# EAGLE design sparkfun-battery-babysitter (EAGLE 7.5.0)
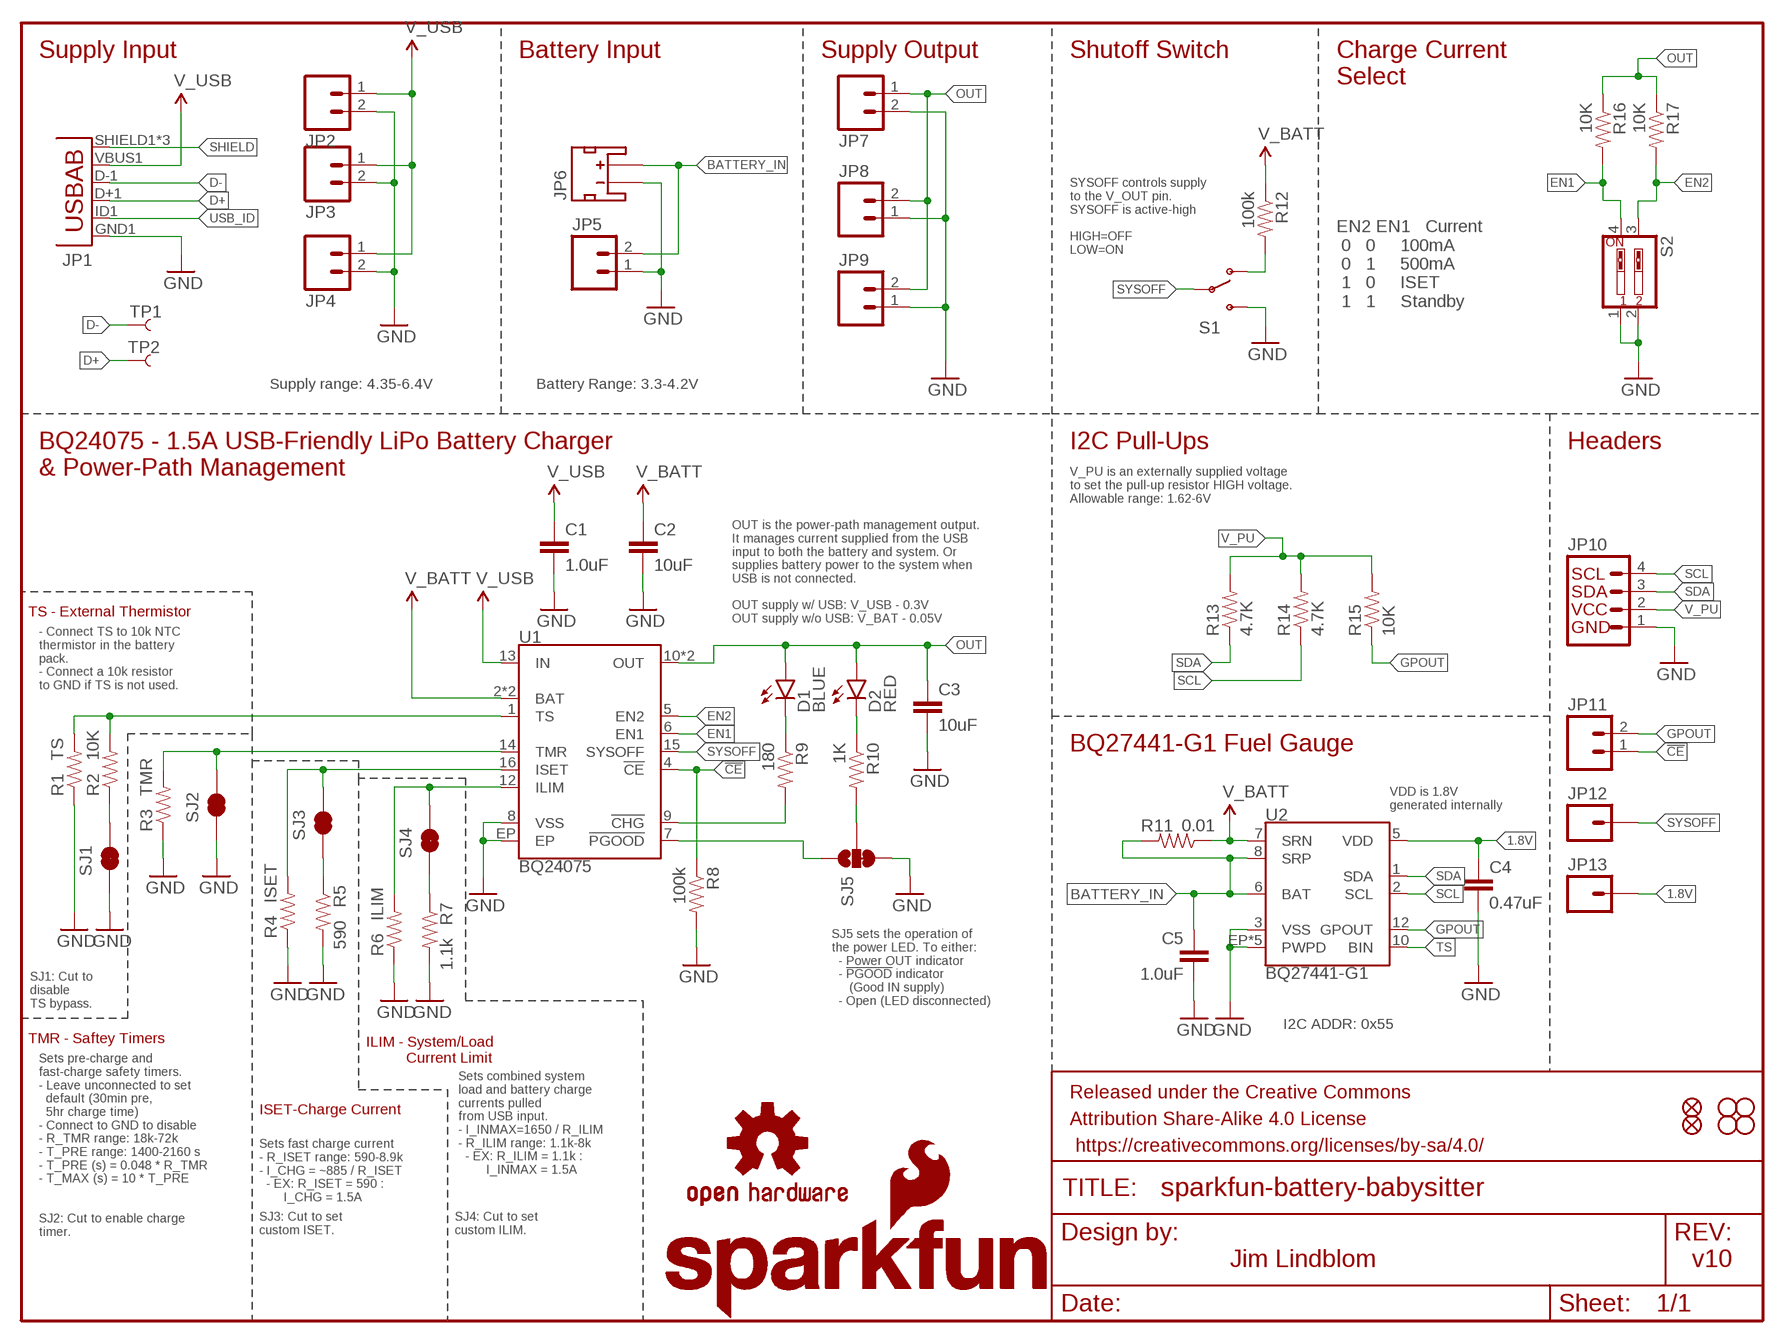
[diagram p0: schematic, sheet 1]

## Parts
C1  1.0uF  1.0UF50V10%(1206)  [1206-CAP]
C2  10uF  10UF10V10%(0805)  [0805-CAP]
C3  10uF  10UF10V10%(0805)  [0805-CAP]
C4  0.47uF  CAP0603-CAP  [0603-CAP]
C5  1.0uF  1.0UF-16V-10%(0603)  [0603-CAP]
D1  BLUE  LED-BLUE0603  [LED-0603]
D2  RED  LED-RED0603  [LED-0603]
FID1  FIDUCIAL1X2  [FIDUCIAL-1X2]
FID2  FIDUCIAL1X2  [FIDUCIAL-1X2]
FRAME1  FRAME-LETTER  [CREATIVE_COMMONS]
JP1  USB-ABCONN-11794  [USB-AB-MICRO-SMD_V03]
JP2  M021X02_NO_SILK  [1X02_NO_SILK]
JP3  M023.5MM-NO_SILK  [SCREWTERMINAL-3.5MM-2-NS]
JP4  M021X02_NO_SILK  [1X02_NO_SILK]
JP5  M021X02_NO_SILK  [1X02_NO_SILK]
JP6  JST_2MM_MALE  [JST-2-SMD]
JP7  M023.5MM-NO_SILK  [SCREWTERMINAL-3.5MM-2-NS]
JP8  M021X02_NO_SILK  [1X02_NO_SILK]
JP9  M02-JST-2-PTH-NO_SILK  [JST-2-PTH-NS]
JP10  I2C_STANDARD_NO_SILK  [1X04_NO_SILK]
JP11  M021X02_NO_SILK  [1X02_NO_SILK]
JP12  M01PTH_NO_SILK_YES_STOP  [1X01_NO_SILK]
JP13  M01PTH_NO_SILK_YES_STOP  [1X01_NO_SILK]
LOGO1  SFE_LOGO_NAME.1_INCH  [SFE_LOGO_NAME_.1]
LOGO2  SFE_LOGO_NAME_FLAME.1_INCH  [SFE_LOGO_NAME_FLAME_.1]
LOGO3  OSHW-LOGOS  [OSHW-LOGO-S]
R1  TS  RESISTORPTH-1/6W  [1/6W-RES]
R2  10K  10KOHM-1/10W-1%(0603)0603  [0603-RES]
R3  TMR  RESISTORPTH-1/6W  [1/6W-RES]
R4  ISET  RESISTORPTH-1/6W  [1/6W-RES]
R5  590  RESISTOR0603-RES  [0603-RES]
R6  ILIM  RESISTORPTH-1/6W  [1/6W-RES]
R7  1.1k  RESISTOR0603-RES  [0603-RES]
R8  100k  100KOHM-1/10W-1%(0603)  [0603-RES]
R9  180  180OHM1/10W1%(0603)  [0603-RES]
R10  1K  1KOHM-1/10W-1%(0603)  [0603-RES]
R11  0.01  RESISTOR1206  [1206]
R12  100k  100KOHM-1/10W-1%(0603)  [0603-RES]
R13  4.7K  4.7KOHM-1/10W-1%(0603)  [0603-RES]
R14  4.7K  4.7KOHM-1/10W-1%(0603)  [0603-RES]
R15  10K  10KOHM-1/10W-1%(0603)0603  [0603-RES]
R16  10K  10KOHM-1/10W-1%(0603)0603  [0603-RES]
R17  10K  10KOHM-1/10W-1%(0603)0603  [0603-RES]
S1  SWITCH-SPDT-SMD-A  [SWITCH-SPST-SMD-A]
S2  SW_DIP-2-SMT-HALFSIZE  [DIPSWITCH-02-50MIL]
SJ1  JUMPER-PAD-2-NC_BY_TRACE  [PAD-JUMPER-2-NC_BY_TRACE_YES_SILK]
SJ2  JUMPER-PAD-2-NC_BY_TRACE  [PAD-JUMPER-2-NC_BY_TRACE_YES_SILK]
SJ3  JUMPER-PAD-2-NC_BY_TRACE  [PAD-JUMPER-2-NC_BY_TRACE_YES_SILK]
SJ4  JUMPER-PAD-2-NC_BY_TRACE  [PAD-JUMPER-2-NC_BY_TRACE_YES_SILK]
SJ5  JUMPER-PAD-3-2OF3_NC_BY_TRACE_SMALL  [PAD-JUMPER-3-2OF3_NC_BY_TRACE_YES_SILK_FULL_BOX]
STANDOFF1  STAND-OFF  [STAND-OFF]
STANDOFF2  STAND-OFF  [STAND-OFF]
STANDOFF3  STAND-OFF  [STAND-OFF]
STANDOFF4  STAND-OFF  [STAND-OFF]
TP1  TEST-POINT3X4  [PAD.03X.04]
TP2  TEST-POINT3X4  [PAD.03X.04]
U1  BQ24075  [PVQFN-N16]
U2  BQ27441-G1  [PDSO-N12]

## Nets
1.8V: C4.1 JP13.1 U2.5(VDD)
!CE!: JP11.1 R8.1 U1.4(!CE!)
!CHG!: R9.2 U1.9(!CHG!)
!PGOOD!: SJ5.1 U1.7(!PGOOD!)
BATTERY_IN: C5.1 JP5.2 JP6.2(+) R11.2 U2.6(BAT) U2.8(SRP)
D+: JP1.D+1(D+) TP2.P$1
D-: JP1.D-1(D-) TP1.P$1
EN1: R16.2 S2.4 U1.6(EN1)
EN2: R17.2 S2.3 U1.5(EN2)
GND: C1.2 C2.2 C3.2 C4.2 C5.2 JP1.GND1(GND) JP2.2 JP3.2 JP4.2 JP5.1 JP6.1(-) JP7.2 JP8.1 JP9.1 JP10.1 R1.1 R3.1 R4.1 R5.2 R6.1 R7.2 R8.2 S1.3(S) S2.1 S2.2 SJ1.1 SJ2.1 SJ5.3 U1.8(VSS) U1.EP U2.3(VSS) U2.EP1(PWPD) U2.EP2(PWPD) U2.EP3(PWPD) U2.EP4(PWPD) U2.EP(PWPD)
GPOUT: JP11.2 R15.1 U2.12(GPOUT)
ILIM: R6.2 SJ4.2 U1.12(ILIM)
ISET: R4.2 SJ3.2 U1.16(ISET)
N$1: R2.1 SJ1.2
N$2: R7.1 SJ4.1
N$3: R5.1 SJ3.1
N$4: R12.2 S1.1(O)
N$5: R10.2 SJ5.2
N$11: D1.C R9.1
N$12: D2.C R10.1
OUT: C3.1 D1.A D2.A JP7.1 JP8.2 JP9.2 R16.1 R17.1 U1.10(OUT) U1.11(OUT)
SCL: JP10.4 R14.1 U2.2(SCL)
SDA: JP10.3 R13.1 U2.1(SDA)
SHIELD: JP1.SHIELD1(SHIELD) JP1.SHIELD2(SHIELD) JP1.SHIELD3(SHIELD)
SYSOFF: JP12.1 S1.2(P) U1.15(SYSOFF)
TMR: R3.2 SJ2.2 U1.14(TMR)
TS: R1.2 R2.2 U1.1(TS) U2.10(BIN)
USB_ID: JP1.ID1(USBID)
V_BATT: C2.1 R11.1 R12.1 U1.2(BAT) U1.3(BAT) U2.7(SRN)
V_PU: JP10.2 R13.2 R14.2 R15.2
V_USB: C1.1 JP1.VBUS1(VBUS) JP2.1 JP3.1 JP4.1 U1.13(IN)
Unconnected: JP6.NC1(PAD1) JP6.NC2(PAD2)

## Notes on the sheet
- Supply Input | Battery Input | Supply Output | Shutoff Switch
- Charge Current
  Select
- SYSOFF controls supply 
  to the V_OUT pin.
  SYSOFF is active-high
  
  HIGH=OFF
  LOW=ON
- EN2 EN1   Current
   0   0     100mA
   0   1     500mA
   1   0     ISET
   1   1     Standby
- Supply range: 4.35-6.4V | Battery Range: 3.3-4.2V
- BQ24075 - 1.5A USB-Friendly LiPo Battery Charger 
  & Power-Path Management
- I2C Pull-Ups | Headers
- V_PU is an externally supplied voltage 
  to set the pull-up resistor HIGH voltage.
  Allowable range: 1.62-6V
- OUT is the power-path management output.
  It manages current supplied from the USB 
  input to both the battery and system. Or
  supplies battery power to the system when 
  USB is not connected.
  
  OUT supply w/ USB: V_USB - 0.3V
  OUT supply w/o USB: V_BAT - 0.05V
- TS - External Thermistor
- - Connect TS to 10k NTC 
  thermistor in the battery
  pack.
  - Connect a 10k resistor 
  to GND if TS is not used.
- BQ27441-G1 Fuel Gauge
- VDD is 1.8V
  generated internally
- SJ5 sets the operation of 
  the power LED. To either:
    - Power OUT indicator
    - !PGOOD! indicator 
       (Good IN supply)
    - Open (LED disconnected)
- SJ1: Cut to 
  disable
  TS bypass.
- I2C ADDR: 0x55
- TMR - Saftey Timers
- ILIM - System/Load 
            Current Limit
- Sets pre-charge and
  fast-charge safety timers.
  - Leave unconnected to set
    default (30min pre, 
    5hr charge time)
  - Connect to GND to disable
  - R_TMR range: 18k-72k
  - T_PRE range: 1400-2160 s
  - T_PRE (s) = 0.048 * R_TMR
  - T_MAX (s) = 10 * T_PRE
- Sets combined system
  load and battery charge 
  currents pulled
  from USB input.
  - I_INMAX=1650 / R_ILIM
  - R_ILIM range: 1.1k-8k
    - EX: R_ILIM = 1.1k : 
          I_INMAX = 1.5A
- ISET-Charge Current
- Sets fast charge current
  - R_ISET range: 590-8.9k
  - I_CHG = ~885 / R_ISET
    - EX: R_ISET = 590 : 
         I_CHG = 1.5A
- SJ3: Cut to set
  custom ISET.
- SJ4: Cut to set
  custom ILIM.
- SJ2: Cut to enable charge
  timer.
- Jim Lindblom | v10

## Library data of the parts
C1 = SparkFun-Capacitors:1.0UF50V10%(1206): CAP-09822; PROD_ID: CAP-09822
C2 C3 = SparkFun-Capacitors:10UF10V10%(0805): CAP-11330; PROD_ID: CAP-11330
C4 = SparkFun-Capacitors:CAP: Capacitor; PROD_ID: CAP-13216
C5 = SparkFun-Capacitors:1.0UF-16V-10%(0603): CAP-00868; PROD_ID: CAP-00868
D1 = SparkFun-LED:LED-BLUE: Blue LEDs for production use; PROD_ID: DIO-08575
D2 = SparkFun-LED:LED-RED: Assorted Red LEDs; PROD_ID: DIO-00819
FID1 FID2 = SparkFun-Aesthetics:FIDUCIAL: Fiducial Alignment Points
FRAME1 = SparkFun-Aesthetics:FRAME-LETTER: Schematic Frame
JP1 = SparkFun-Connectors:USB-AB: This is a USB AB connector that is compatible with USB OTG. i.e. this connector can serve as a host or device; PROD_ID: CONN-11794
JP2 JP4 JP5 JP8 JP9 JP11 = SparkFun-Connectors:M02: Standard 2-pin 0.1" header. Use with
JP3 JP7 = SparkFun-Connectors:M02: Standard 2-pin 0.1" header. Use with; PROD_ID: CONN-08399
JP6 = SparkFun-Connectors:JST_2MM_MALE: Mates to single-cell LiPo batteries. CONN-11443 Now with smashable polarity marks!; BTM_NEG: -; BTM_POS: +; PROD_ID: CONN-11443; TOP_NEG: -; TOP_POS: +
JP10 = SparkFun-Connectors:I2C_STANDARD: SparkFun has standardized on a pinout for all I2C based sensor breakouts. This pinout allows I2C boards to be plugged directly into the headers on Arduino Uno compatible boards, and to be daisy chained easily.
JP12 JP13 = SparkFun-Connectors:M01: Header 1
LOGO1 = SparkFun-Aesthetics:SFE_LOGO_NAME: SFE Logo, name only
LOGO2 = SparkFun-Aesthetics:SFE_LOGO_NAME_FLAME: SFE Logo, name and flame
LOGO3 = SparkFun-Aesthetics:OSHW-LOGO: Open Source Hardware Logo
R1 R3 R4 R6 = SparkFun-Resistors:RESISTOR: Resistor
R2 R15-R17 = SparkFun-Resistors:10KOHM-1/10W-1%(0603): RES-00824; PROD_ID: RES-00824
R5 = SparkFun-Passives:RESISTOR: Resistor; PROD_ID: RES-13217
R7 = SparkFun-Passives:RESISTOR: Resistor; PROD_ID: RES-10447
R8 R12 = SparkFun-Resistors:100KOHM-1/10W-1%(0603): RES-07828; PROD_ID: RES-07828
R9 = SparkFun-Resistors:180OHM1/10W1%(0603): RES-08788; PROD_ID: RES-08788
R10 = SparkFun-Resistors:1KOHM-1/10W-1%(0603): RES-07856; PROD_ID: RES-07856
R11 = SparkFun-Resistors:RESISTOR: Resistor; PROD_ID: RES-13218
R13 R14 = SparkFun-Resistors:4.7KOHM-1/10W-1%(0603): RES-07857; PROD_ID: RES-07857
S1 = SparkFun-Electromechanical:SWITCH-SPDT: SPDT Switch Simple slide switch, Spark Fun Electronics SKU : COM-00102 DPDT SMT slide switch, AYZ0202, SWCH-08179; PROD_ID: SWCH-10651
S2 = SparkFun-Electromechanical:SW_DIP-2: DIP SWITCH; PROD_ID: SWCH-13215
SJ1-SJ4 = SparkFun-Passives:JUMPER-PAD-2-NC_BY_TRACE
SJ5 = SparkFun-Passives:JUMPER-PAD-3-2OF3_NC_BY_TRACE
STANDOFF1-STANDOFF4 = SparkFun-Electromechanical:STAND-OFF: #4 Stand Off
TP1 TP2 = SparkFun-Passives:TEST-POINT: Bare copper test points for troubleshooting or ICT
U1 = battery-management-temp:BQ24075; PROD_ID: IC-13219
U2 = battery-management-temp:BQ27441-G1; PROD_ID: IC-13220

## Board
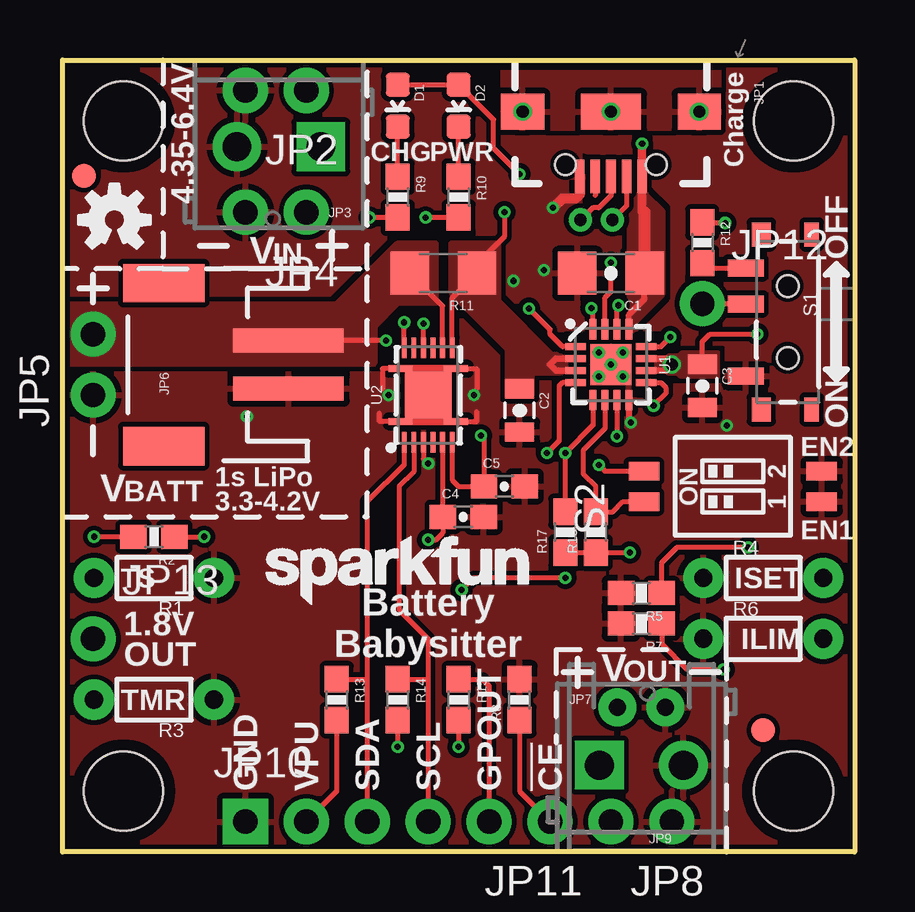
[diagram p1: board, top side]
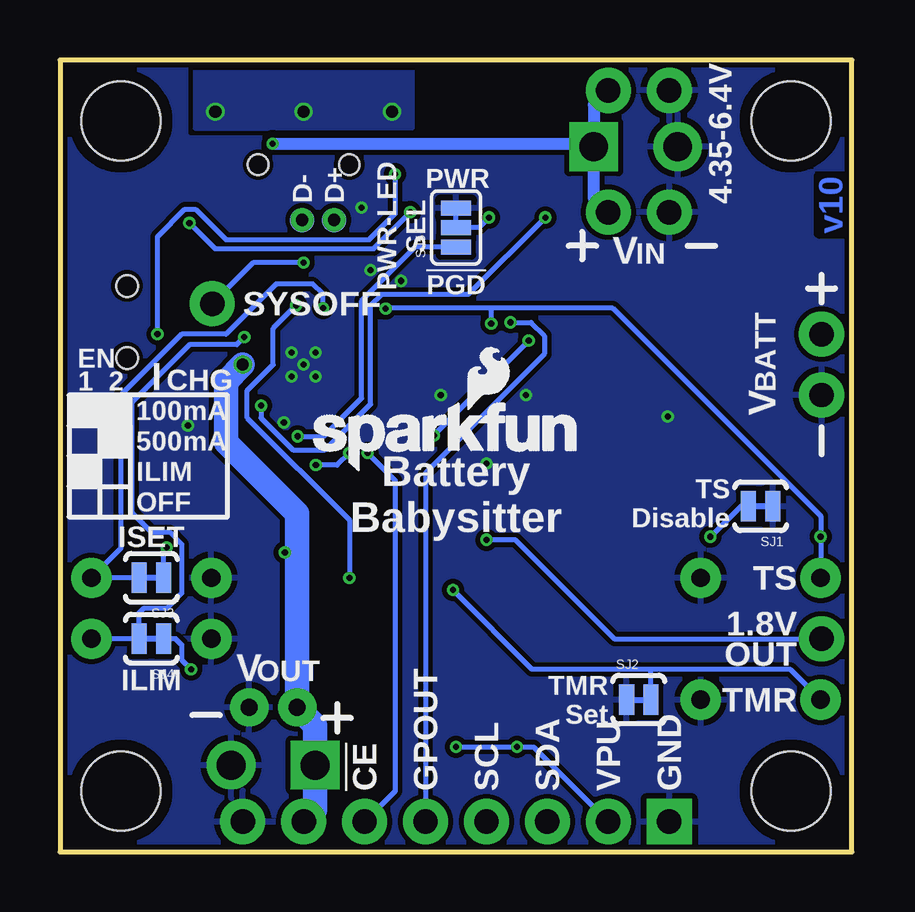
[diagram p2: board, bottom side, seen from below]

Size 33.02 x 33.02 mm. Coordinates in mm from the lower left corner, seen from the top.
Outline: 0,33.02 33.02,33.02 33.02,0 0,0 0,33.02
Copper layers (1*16): Top 0.035mm / dielectric 1.5mm / Bottom 0.035mm
Design rules "SparkFun-2-layer-FAB-LIMIT *": minimum track width 7mil, minimum drill 6mil, track to track 7mil, track to pad 7mil, pad to pad 7mil, via to via 7mil, smd to smd 7mil, copper to edge 7mil, drill to drill 7mil, minimum pad ring 5mil, minimum via ring 5mil, stop-mask expansion 4mil, vias tented up to drill 20mil, thermal gap 10mil

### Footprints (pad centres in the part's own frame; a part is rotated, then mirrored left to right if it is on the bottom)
1206-CAP = smd 1.6 x 1.8: 1 -1.4,0; 2 1.4,0
0805-CAP = smd 0.8 x 1.2: 1 -0.9,0; 2 0.9,0
0603-CAP = smd 1.1 x 1: 1 -0.85,0; 2 0.85,0
LED-0603 = smd 1 x 1: A 0,-0.877; C 0,0.877
FIDUCIAL-1X2 = smd 1 x 1: 1 0,0
USB-AB-MICRO-SMD_V03 = smd 1.4 x 0.4: D+1 2.7,0; D-1 2.7,0.65; GND1 2.7,-1.3; ID1 2.7,-0.65; VBUS1 2.7,1.3 | smd 1.5 x 1.8: SHIELD1 0,3.68; SHIELD3 0,-3.68 | smd 1.5 x 2.5: SHIELD2 0,0 | hole 0.85: 2.2,1.9; 2.2,-1.9
1X02_NO_SILK = drill 1.016 pad 1.88: 1 0,0; 2 2.54,0
SCREWTERMINAL-3.5MM-2-NS = drill 1.2 pad 2.032 square: 1 0,0 | drill 1.2 pad 2.032: 2 3.5,0
JST-2-SMD = smd 1 x 4.6: 1 -1,-3.7; 2 1,-3.7 | smd 1.6 x 3.4: NC1 -3.4,1.5; NC2 3.4,1.5
JST-2-PTH-NS = drill 0.7 pad 1.6: 1 -1,0; 2 1,0
1X04_NO_SILK = drill 1.016 pad 1.88 square: 1 0,0 | drill 1.016 pad 1.88: 2 2.54,0; 3 5.08,0; 4 7.62,0
1X01_NO_SILK = drill 1.016 pad 1.88: 1 0,0
1/6W-RES = drill 0.762 pad 1.676: 1 -2.5,0; 2 2.5,0
0603-RES = smd 1.1 x 1: 1 -0.85,0; 2 0.85,0
1206 = smd 1.6 x 1.8: 1 -1.4,0; 2 1.4,0
SWITCH-SPST-SMD-A = smd 0.7 x 1.5: 1 -2.25,-1.75; 2 -0.75,-1.75; 3 2.25,-1.75 | smd 1 x 0.6: GND1 -3.65,1; GND3 3.65,1 | smd 1 x 0.8: GND2 -3.65,-1.1; GND4 3.65,-1.1 | hole 0.9: -1.5,0; 1.5,0
DIPSWITCH-02-50MIL = smd 0.762 x 1.27: 1 -0.635,-3.7; 2 0.635,-3.7; 3 0.635,3.7; 4 -0.635,3.7
PAD-JUMPER-2-NC_BY_TRACE_YES_SILK = smd 0.635 x 1.27: 1 -0.508,0; 2 0.508,0
PAD-JUMPER-3-2OF3_NC_BY_TRACE_YES_SILK_FULL_BOX = smd 0.635 x 1.27: 1 -0.813,0; 2 0,0; 3 0.813,0
STAND-OFF = hole 3.302: 0,0
PAD.03X.04 = smd 1.016 x 1.016: P$1 0,0
PVQFN-N16 = smd 0.28 x 0.85: 1 -0.75,-1.475; 2 -0.25,-1.475; 3 0.25,-1.475; 4 0.75,-1.475; 9 0.75,1.475; 10 0.25,1.475; 11 -0.25,1.475; 12 -0.75,1.475 | smd 0.85 x 0.28: 5 1.475,-0.75; 6 1.475,-0.25; 7 1.475,0.25; 8 1.475,0.75; 13 -1.475,0.75; 14 -1.475,0.25; 15 -1.475,-0.25; 16 -1.475,-0.75 | smd 1.7 x 1.7: EP 0,0
PDSO-N12 = smd 0.2 x 0.85: 1 -1,-1.975; 2 -0.6,-1.975; 3 -0.2,-1.975; 4 0.2,-1.975; 5 0.6,-1.975; 6 1,-1.975; 7 1,1.975; 8 0.6,1.975; 9 0.2,1.975; 10 -0.2,1.975; 11 -0.6,1.975; 12 -1,1.975 | smd 1.95 x 1.95: EP 0,0 | smd 1 x 0.25: EP1 -1.15,1.1; EP2 -1.15,-1.1; EP3 1.15,-1.1; EP4 1.15,1.1

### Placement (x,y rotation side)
C1  22.86,24.13 180 top
C2  19.05,18.41 270 top
C3  26.67,19.43 270 top
C4  16.7,13.97 0 top
C5  18.41,15.24 0 top
D1  13.97,31.11 180 top
D2  16.51,31.11 180 top
FID1  0.89,28.19 0 top
FID2  29.21,5.08 0 top
FRAME1  not placed on the board
JP1  22.86,30.86 270 top
JP2  10.16,31.75 180 top
JP3  10.77,29.4 180 top
JP4  10.16,26.67 180 top
JP5  1.27,19.05 90 top
JP6  5.71,20.32 90 top
JP7  22.38,3.62 0 top
JP8  25.4,1.27 180 top
JP9  24.13,6.03 180 top
JP10  7.62,1.27 0 top
JP11  20.32,1.27 180 top
JP12  26.67,22.86 0 top
JP13  1.27,8.89 0 top
LOGO1  8,9.84 0 top
LOGO2  22.86,15.81 0 bottom
LOGO3  2.16,26.35 0 top
R1  3.81,11.43 180 top
R2  3.81,13.14 180 top
R3  3.81,6.35 180 top
R4  29.21,11.43 0 top
R5  24.13,10.79 180 top
R6  29.21,8.89 0 top
R7  24.13,9.53 180 top
R8  19.05,6.35 90 top
R9  13.97,27.3 270 top
R10  16.51,27.3 270 top
R11  15.88,24.13 180 top
R12  26.67,25.4 270 top
R13  11.43,6.35 270 top
R14  13.97,6.35 270 top
R15  16.51,6.35 270 top
R16  22.23,13.34 90 top
R17  20.95,13.34 90 top
S1  30.23,22.1 270 top
S2  27.94,15.24 90 top
SJ1  3.81,14.41 180 bottom
SJ2  8.89,6.35 0 bottom
SJ3  29.21,11.43 180 bottom
SJ4  29.21,8.89 180 bottom
SJ5  16.51,26.04 90 bottom
STANDOFF1  30.48,30.48 0 top
STANDOFF2  2.54,2.54 0 top
STANDOFF3  2.54,30.48 0 top
STANDOFF4  30.48,2.54 0 top
TP1  22.92,26.35 0 bottom
TP2  21.59,26.35 0 bottom
U1  22.86,20.32 270 top
U2  15.24,19.05 0 top

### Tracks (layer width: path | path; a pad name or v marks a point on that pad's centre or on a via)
1.8V  (via drill 0.25)
  Top 0.203: U2.5 C4.1 15.85,13.31 15.56,13.02 v15.24,13.02
  Bottom 0.203: JP13.1 9.91,8.89 14.03,13.02 v15.24,13.02
!CE!  (via drill 0.25)
  Top 0.203: U1.4 20.84,19.57 20.7,19.43 20.7,17.14 v20.19,16.64 | R8.1 19.05,2.54 JP11.1
  Bottom 0.203: v20.19,16.64 19.05,15.49 19.05,2.54 JP11.1
!CHG!  (via drill 0.25)
  Top 0.203: U1.9 24.94,19.57 25.15,19.37 25.15,19.11 v24.64,18.61 | R9.2 v12.79,26.45
  Bottom 0.203: v24.64,18.61 24.64,18.1 23.3,16.76 21.97,16.76 20.07,18.67 20.07,22.8 19.62,23.24 16,23.24 v12.79,26.45
!PGOOD!  (via drill 0.25)
  Top 0.203: U1.7 v23.11,17.33
  Bottom 0.203: v23.11,17.33 22.04,17.33 20.45,18.92 20.45,22.99 18.21,25.22 SJ5.1
BATTERY_IN  (via drill 0.25)
  Top 0.203: U2.8 15.84,22.77 R11.2 | U2.6 16.24,15.51 16.51,15.24 C5.1 17.57,17.23 v17.44,17.36 | v13.48,21.32 JP6.2
  Bottom 0.203: v13.48,21.32 v17.44,17.36
  pour Top (isolate 0.203, no thermals): 0,22.86 11.43,22.86 13.97,25.4 15.56,25.4 15.56,22.86 13.97,22.86 13.02,21.91 13.02,20.32 0,20.32
D+  (via drill 0.51 pad 0.97)
  Top 0.203: JP1.D+1 22.86,27.37 22.35,26.86 22.1,26.86 TP2.P$1
  other vias: 21.59,26.35
D-  (via drill 0.51 pad 0.97)
  Top 0.203: JP1.D-1 23.51,26.94 TP1.P$1
  other vias: 22.92,26.35
EN1
  Top 0.203: U1.6 22.61,17.66 21.72,16.76 21.72,15.75 22.23,15.24 R16.2 22.95,14.19 23.37,14.61 S2.4
EN2  (via drill 0.25)
  Top 0.203: U1.5 22.11,17.79 v20.95,16.64 R17.2 | v22.35,16.13 22.61,15.88 S2.3
  Bottom 0.203: v20.95,16.64 21.46,16.13 v22.35,16.13
GND  (via drill 0.25)
  Top 0.203: U2.EP1 13.34,20.15 13.34,19.3 | U2.EP4 17.27,20.15 17.27,19.3 | U2.EP3 17.27,17.95 17.27,18.35 | U2.EP2 13.21,17.95 13.21,18.29 | U2.3 15.04,16.39 v15.24,16.19
  Top 0.254: U2.EP1 15.24,20.15 | U1.8 23.61,18.11
  Top 0.406: JP1.GND1 21.56,27.4 21.4,27.24 20.83,27.24 v20.45,26.86
  other vias: 22.86,20.32 23.36,20.82 23.36,19.82 22.36,19.82 22.36,20.82 17.14,19.05 13.59,19.05 23.69,17.91 20.07,24.26 7.68,18.16 27.69,17.78 18.8,23.81
  pour Top (isolate 0.203, rank 6): 0,33.02 0,0 33.02,0 33.02,33.02
  pour Bottom (isolate 0.203, rank 6): 0,33.02 0,0 33.02,0 33.02,33.02
GPOUT  (via drill 0.25)
  Top 0.203: U2.12 v14.24,22.08 | R15.1 17.5,7.2 17.78,6.92 JP11.2
  Bottom 0.203: v14.24,22.08 13.38,22.08 12.83,21.53 12.83,20.77 17.78,15.81 JP11.2
ILIM  (via drill 0.25)
  Top 0.203: U1.12 24.94,21.07 v25.34,21.46
  Bottom 0.203: v25.34,21.46 25.65,21.14 27.62,21.14 30.04,18.73 30.04,14.16 29.21,13.34 28.45,13.34 27.94,12.83 27.94,10.79 28.57,10.16 29.53,10.16 29.72,9.97 SJ4.2 R6.2
ISET  (via drill 0.25)
  Top 0.203: U1.16 22.11,22.61 v22.05,22.67
  Bottom 0.203: SJ3.2 R4.2 30.48,12.66 30.48,19.05 27.94,21.59 26.1,21.59 24,23.69 22.48,23.69 22.05,23.25 v22.05,22.67
N$1  (via drill 0.25)
  Top 0.203: R2.1 v5.91,13.14
  Bottom 0.203: v5.91,13.14 4.64,14.41 SJ1.2
N$2  (via drill 0.25)
  Top 0.203: R7.1 24.98,8.68 26.04,7.62 v27.56,7.62
  Bottom 0.203: SJ4.1 28.19,8.89 27.94,8.64 27.94,8 v27.56,7.62
N$3  (via drill 0.25)
  Top 0.203: v28.57,12.7 25.61,12.7 24.98,12.06 R5.1
  Bottom 0.203: SJ3.1 28.7,12.57 v28.57,12.7
N$4
  Top 0.203: 27.94,24.55 28.27,24.55 S1.1 26.87,24.35 R12.2
N$5  (via drill 0.25)
  Top 0.203: R10.2 v15.14,26.45
  Bottom 0.203: v15.14,26.45 15.56,26.04 SJ5.2
N$11
  Top 0.203: R9.1 D1.C
N$12
  Top 0.203: R10.1 D2.C
OUT  (via drill 0.25, 0.51)
  Top 0.203: R17.1 R16.1 v23.65,12.48 | C3.1 26.67,21.27 26.99,21.59 v28.96,21.59 | v19.05,28.26 17.97,29.34 17.97,30.53 D2.A D1.A
  Top 0.279: U1.11 25.15,20.57 v25.4,20.32 25.15,20.07 U1.10
  Bottom 0.203: 23.13,11.43 23.13,10.16 23.13,9.65 | v28.96,21.59 28.96,25.65 27.81,26.8 27.37,26.8 26.1,25.53 20.13,25.53 19.05,26.61 v19.05,28.26 | v23.65,12.48 23.13,12.48
  Bottom 1.016: JP8.2 22.38,1.75 JP7.1 22.38,5.28 JP9.2 23.13,10.16 23.13,12.48 23.13,14.11 26.1,17.08 26.1,19.62 v25.4,20.32
  pour Top (isolate 0.305, no thermals): 24.77,20.7 25.72,20.7 25.84,20.83 27.3,20.83 27.3,19.81 25.78,19.81 25.65,19.94 24.77,19.94
SCL
  Top 0.203: 15.24,7.2 15.24,8.89 14.03,10.1 14.03,15.24 14.64,15.85 U2.2 | 15.24,7.2 JP10.4 | R14.1 15.24,7.2
SDA
  Top 0.203: U2.1 14.24,16.14 12.7,14.61 12.7,7.2 | 12.7,7.2 JP10.3 | R13.1 12.7,7.2
SHIELD  (via drill 0.51)
  other vias: 19.18,30.86 26.54,30.86 22.86,30.86
  pour Bottom (isolate 0.305): 18.35,33.02 18.35,30.16 27.37,30.16 27.37,33.02
  pour Top (isolate 0.305): 27.37,33.02 27.37,30.16 18.35,30.16 18.35,33.02
SYSOFF  (via drill 0.25)
  Top 0.203: v22.86,24.57 22.86,23.36 22.61,23.11 U1.15 | JP12.1 28.46,22.86 S1.2
  Bottom 0.203: v22.86,24.57 24.96,24.57 JP12.1
TMR  (via drill 0.25)
  Top 0.203: v20.95,11.43 17.14,11.43 v16.64,10.92 | U1.14 23.11,22.73 v23.17,22.79
  Bottom 0.203: v23.17,22.79 24.13,21.84 24.13,20.32 25.21,19.24 25.21,18.1 20.95,13.84 v20.95,11.43 | 8.38,7.62 2.58,7.62 R3.2 | 8.38,7.62 13.34,7.62 v16.64,10.92 | SJ2.2 8.38,7.62
TS  (via drill 0.25)
  Top 0.203: U2.10 v15.04,22.02 | U1.1 20.84,21.07 20.32,21.59 20.32,21.78 v19.44,22.66 | R2.2 v1.31,13.14
  Bottom 0.203: 15.04,22.67 9.97,22.67 1.31,14.01 v1.31,13.14 R1.2 | 15.04,22.67 v19.43,22.67 v19.44,22.66 | v15.04,22.02 15.04,22.67
USB_ID
  Top 0.203: JP1.ID1 22.21,27.37
V_BATT  (via drill 0.25)
  Top 0.203: U2.7 16.24,23.09 R11.1 17.27,24.51 18.41,25.65 v18.41,26.67 | v27.62,26.23 26.7,26.23 R12.1
  Top 0.279: U1.2 20.57,20.57 20.32,20.32 20.57,20.07 U1.3
  Bottom 0.203: v27.62,26.23 26.54,25.15 19.94,25.15 v18.41,26.67
  pour Top (isolate 0.203, no thermals): 16.19,25.4 18.16,25.4 18.16,22.99 20.38,20.76 20.95,20.76 20.95,19.94 19.56,19.94 19.56,19.05 18.54,19.05 18.54,20.95 16.19,23.3
V_PU  (via drill 0.25)
  Top 0.203: R13.2 11.43,2.54 JP10.2 | R14.2 v13.97,4.38 | R15.2 v16.51,4.38
  Bottom 0.203: JP10.2 13.27,4.38 v13.97,4.38 v16.51,4.38
V_USB  (via drill 0.25)
  Top 0.254: U1.13 23.61,22.4 24.26,23.05 C1.1
  Top 0.356: 24.16,26.67 JP1.VBUS1 v24.16,29.53
  Top 0.508: 24.26,26.67 C1.1
  Bottom 0.508: v24.16,29.53 10.89,29.53 JP3.1 | JP2.1 10.77,31.14 JP3.1 | JP4.1 10.77,27.28 JP3.1
  pour Top (isolate 0.203, no thermals): 23.62,21.46 23.62,27.05 24,27.43 24.32,27.43 25.02,26.73 25.02,23.24 23.88,22.1 23.88,21.46

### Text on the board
Bottom: v10
tPlace: 4.35-6.4V | Charge | CHG | PWR | V | IN | OFF | ON | EN2 | 1s LiPo | V | BATT | 3.3-4.2V | EN1 | Battery / Babysitter | 1.8V | OUT | V | OUT | GND | VPU | SDA | SCL | GPOUT | !CE!
bPlace: 4.35-6.4V | PWR | D+ | D- | PWR-LED / SEL | IN | V | !PGD! | SYSOFF | EN | BATT | V | CHG | I | 2 | 1 | 100mA | Battery / Babysitter | 500mA | ILIM | TS / Disable | OFF | ISET | TS | 1.8V | OUT | ILIM | OUT | V | TMR | TMR / Set | GND | VPU | SDA | SCL | GPOUT | !CE!
Measures: Units in inches
tDocu: Jim Lindblom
